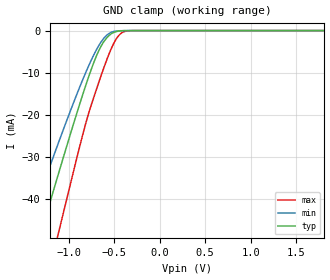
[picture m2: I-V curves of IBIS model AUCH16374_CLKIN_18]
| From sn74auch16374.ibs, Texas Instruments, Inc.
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[Model]   AUCH16374_CLKIN_18
Model_type  Input
Vinl=0.5775
Vinh=1.2675
| variable   typ   min   max
C_comp   2.44pF   2.00pF   2.78pF
[Temperature Range]   40   100   -40
| Ambient temperature   25   85   -40
[Voltage range]   1.8   1.65   1.95
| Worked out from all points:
|   GND clamp passes 1 mA (typ) near -0.55 V on its own axis
[GND Clamp]
| AUCH16374_CLKIN_18
|   Voltage   I(typ)   I(min)   I(max)
-3.6V     -222.3mA   -186.1mA   -267.5mA
-1.475V   -61.16mA   -48.85mA   -80.77mA
-1.43V    -57.79mA   -46.07mA   -76.76mA
-1.295V   -47.7mA    -37.79mA   -64.71mA
-1.145V   -36.62mA   -28.76mA   -51.31mA
-1.095V   -32.97mA   -25.81mA   -46.85mA
-830mV    -14.31mA   -10.96mA   -23.64mA
-685mV    -5.607mA   -4.224mA   -13.41mA
-560mV    -1.272mA   -753.7uA   -5.827mA
-485mV    -290.6uA   -140.2uA   -2.305mA
-420mV    -55.81uA   -26.72uA   -608.5uA
1.8V      203.2pA    297.2pA    235.5pA
